/// Change the DPS402 mode if 
/// Mode of operation is not equal to Mode of operation Display.
/// 
/// This function block leaves the motor enabled and in Operation 
/// Enable state, if suceeded.
  
FUNCTION_BLOCK MIS_ChangeDSP402mode
VAR_INPUT
	eCmd : eCommand;
	siModeOfOperation : SINT;
END_VAR
VAR_IN_OUT
	stMisMotorLocal : stMisMotor;	
END_VAR
VAR_OUTPUT
	eError : eErrorCodesMIS;
	eStat: ESTATUS;
END_VAR
VAR

	iState: INT;
	MISenableMotori: MIS_EnableMotor;

	bFirstTry: BOOL;
END_VAR

IF eCmd = eCommand.Reset THEN
	MISenableMotori(eCmd := eCommand.Reset,stMisMotorLocal := stMisMotorLocal);
	eError := eErrorCodesMIS.None;
	iState := 0;
	eStat := eStatus.Done;
	RETURN;
END_IF;



CASE iState OF 
0:
	CASE eCmd OF
	eCommand.Run:
		eStat := eStatus.Running;
		eError := eErrorCodesMIS.None;
		iState := 100;
		bFirstTry := TRUE;
	END_CASE

100: //Set state 
	stMisMotorLocal.siModesOfOperation := siModeOfOperation; //Profile position mode
	iState := iState + 1;

101://Enable motor
	MISenableMotori(eCmd := eCommand.Run,bEnable := TRUE,stMisMotorLocal := stMisMotorLocal);
	IF MISenableMotori.eStat = eStatus.Done THEN
		 MISenableMotori(eCmd := eCommand.Reset,stMisMotorLocal := stMisMotorLocal);
		 iState := iState + 1;
	ELSIF MISenableMotori.eStat = eStatus.Error THEN
		eError := eErrorCodesMIS.ModeChangeEnableFailed;
		eStat := eStatus.Error; //Correct mode not optained						
		
	END_IF;
	
102: //Test actual mode 
	IF stMisMotorLocal.siModesOfOperationDisplay = siModeOfOperation THEN
		eStat := eStatus.Done;
		iState := 1000;
	ELSE
		IF bFirstTry THEN 
			bFirstTry := FALSE;
			iState := 110;
		ELSE
			eStat := eStatus.Error; //Correct mode not optained
			eError := eErrorCodesMIS.ModeChangeFailed;						
		END_IF;
	END_IF
	 
110://Disable motor
	MISenableMotori(eCmd := eCommand.Run,bEnable := FALSE,stMisMotorLocal := stMisMotorLocal);
	IF MISenableMotori.eStat = eStatus.Done THEN
		 MISenableMotori(eCmd := eCommand.Reset,stMisMotorLocal := stMisMotorLocal);
		 iState := 100; //try again
	 ELSE
		eStat := eStatus.Error; //Correct mode not optained
		eError := eErrorCodesMIS.ModeChangeDisableFailed;						
	END_IF;

	

1000: //Done witout error

END_CASE

END_FUNCTION_BLOCK
